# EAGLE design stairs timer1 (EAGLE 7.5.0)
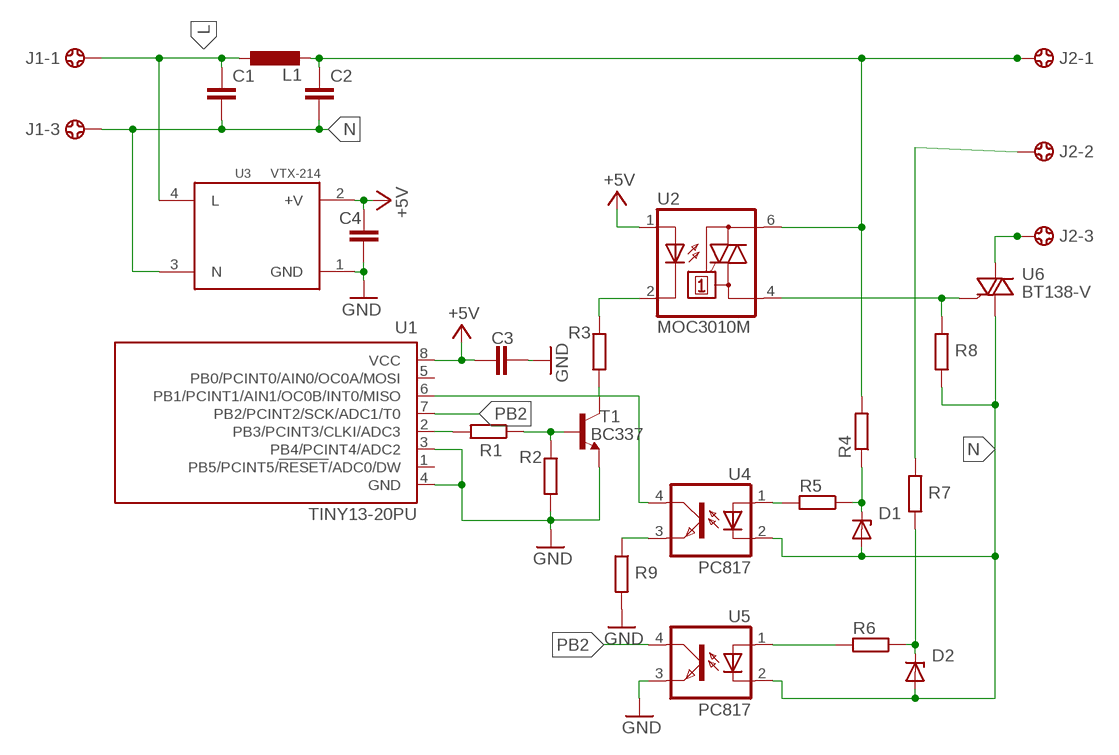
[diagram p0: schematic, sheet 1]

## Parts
C1  C-EU150-072X183  [C150-072X183]
C2  C-EU150-072X183  [C150-072X183]
C3  C-EUC1206  [C1206]
C4  C-EUC1206  [C1206]
D1  1N4728  [DO41Z10]
D2  1N4728  [DO41Z10]
J1  5202-03-N-02  [5202-03-N-02]
J2  5202-03-N-02  [5202-03-N-02]
L1  L-EUTJ8-U1  [TJ8-U1]
R1  R-EU_0204/7  [0204/7]
R2  R-EU_0204/7  [0204/7]
R3  R-EU_0204/7  [0204/7]
R4  R-EU_0617/22  [0617/22]
R5  R-EU_0204/7  [0204/7]
R6  R-EU_0204/7  [0204/7]
R7  R-EU_0617/22  [0617/22]
R8  R-EU_0204/7  [0204/7]
R9  R-EU_0204/7  [0204/7]
T1  BC337  [TO92]
U1  TINY13-20PU  [DIL08]
U2  MOC3010M  [DIL06]
U3  VTX-214  [VTX-214]
U4  PC817  [DIL04]
U5  PC817  [DIL04]
U6  BT138-V  [TO220BV]

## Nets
+5V: C3.1 C4.1 U1.8(VCC) U2.1(A) U3.2(+V)
GND: C3.2 C4.2 R2.2 R9.2 T1.1(E) U1.3(PB4/PCINT4/ADC2) U1.4(GND) U3.1(GND) U5.3(EMIT)
L: C1.1 J1.1 L1.1 U3.4(L)
N: C1.2 C2.2 D1.A D2.A J1.3 R8.2 U3.3(N) U4.2(C) U5.2(C) U6.T1(A1)
N$1: R1.2 U1.2(PB3/PCINT3/CLKI/ADC3)
N$2: R1.1 R2.1 T1.2(B)
N$3: C2.1 J2.1 L1.2 R4.2 U2.6(A2)
N$4: R5.2 U4.1(A)
N$5: R3.2 T1.3(C)
N$6: R3.1 U2.2(C)
N$7: D1.C R4.1 R5.1
N$8: R6.2 U5.1(A)
N$9: D2.C R6.1 R7.1
N$10: J2.2 R7.2
N$11: R8.1 U2.4(A1) U6.G
N$12: J2.3 U6.T2(A2)
N$13: R9.1 U4.3(EMIT)
PB1: U1.6(PB1/PCINT1/AIN1/OC0B/INT0/MISO) U4.4(COL)
PB2: U1.7(PB2/PCINT2/SCK/ADC1/T0) U5.4(COL)
Unconnected: J1.2 U1.1(PB5/PCINT5/!RESET!/ADC0/DW) U1.5(PB0/PCINT0/AIN0/OC0A/MOSI)

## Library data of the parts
C1-C4 = rcl:C-EU: CAPACITOR, European symbol
D1 D2 = diode:1N4728: Z DIODE
J1 J2 = con-ebyelectro:5202-03-N-02: Barrier Blocks Sreies 5202 Source: http://www.ebyelectro.com/PDF/5202-XX-N-02.pdf; OC_FARNELL: unknown; OC_NEWARK: unknown
L1 = rcl:L-EU: INDUCTOR, European symbol
R1-R9 = rcl:R-EU_: RESISTOR, European symbol
T1 = transistor:BC337: NPN TRANSISTOR
U1 = atmel:TINY13: 8-bit AVR Microcontroller with 1K Bytes In-System Programmable Flash Source: http://www.atmel.com/dyn/resources/prod_documents/2535S.pdf; MPN: ATTINY13-20PU; OC_FARNELL: 9171550; OC_NEWARK: 96K6521
U2 = optocoupler:MOC30*M: RANDOM-PHASE OPTOISOLATORS TRIAC DRIVER OUTPUT Source: http://www.fairchildsemi.com MOC3020-M.pdf; MF: FAIRCHILD SEMICONDUCTOR; MPN: MOC3010-M; OC_FARNELL: 1505423; OC_NEWARK: 72K8892
U3 = acdc:VTX-214: ACDC CONVERTER
U4 U5 = optocoupler:PC817: SHARP OPTO COUPLER; MPN: PC817X4J000F; OC_FARNELL: 9707727; OC_NEWARK: 97K7059
U6 = triac:BT138: TRIAC Source: http://www.semiconductors.philips.com BT138_SERIES_2.pdf

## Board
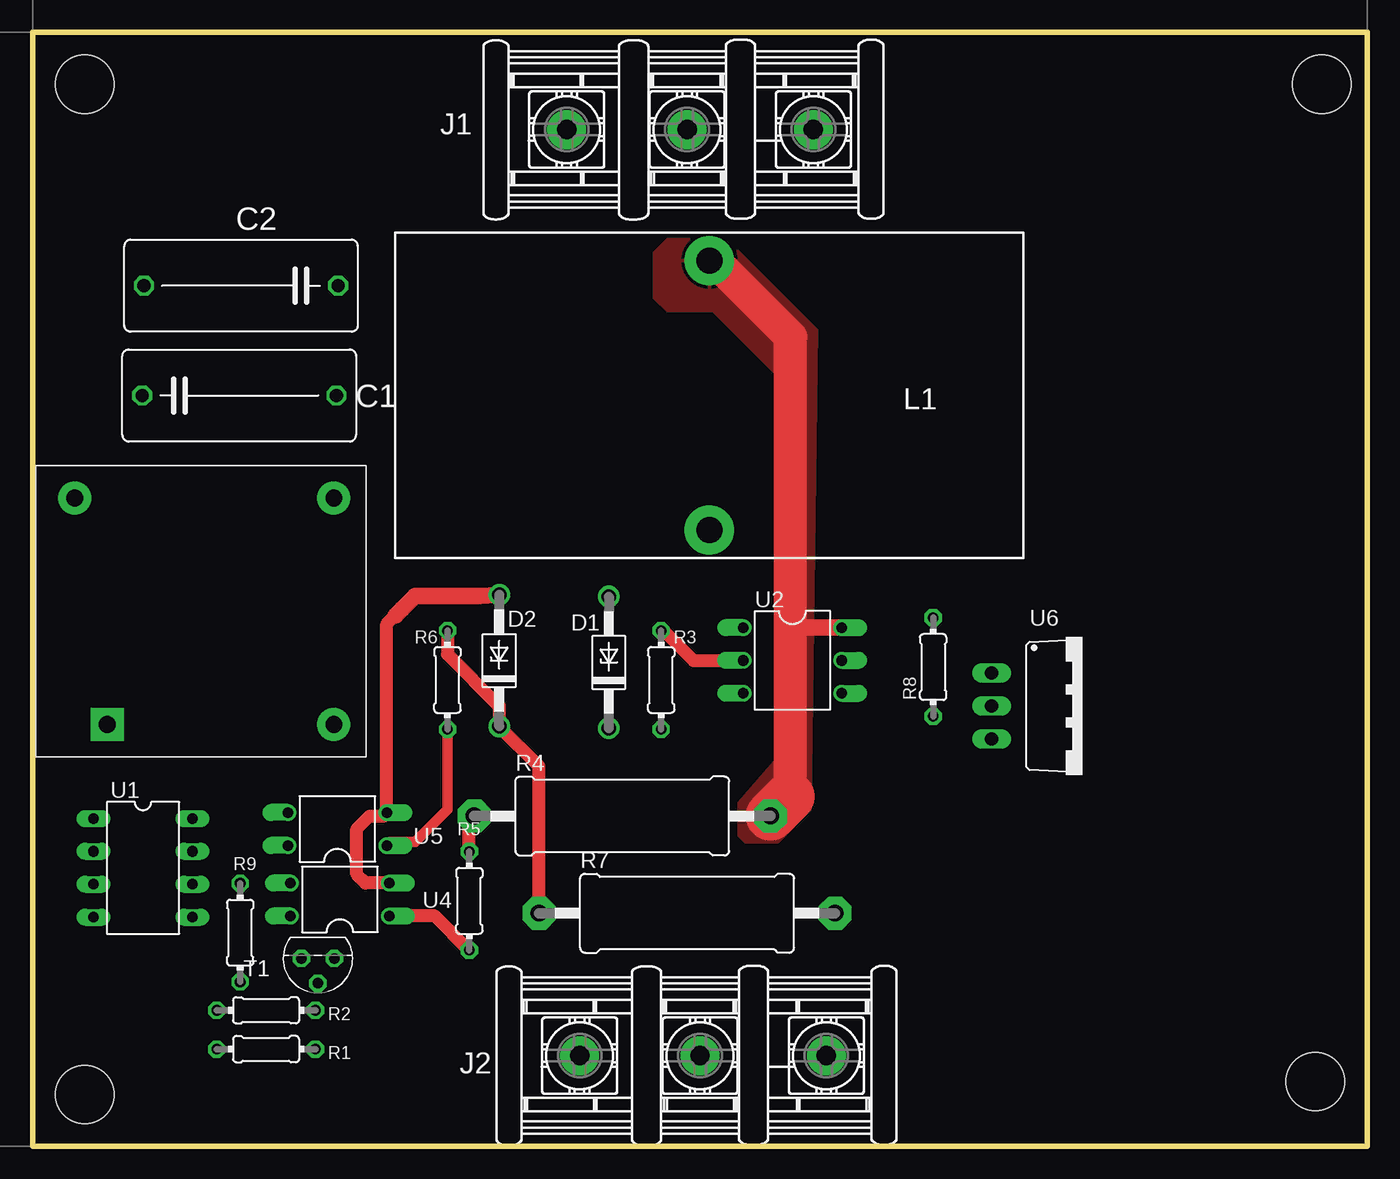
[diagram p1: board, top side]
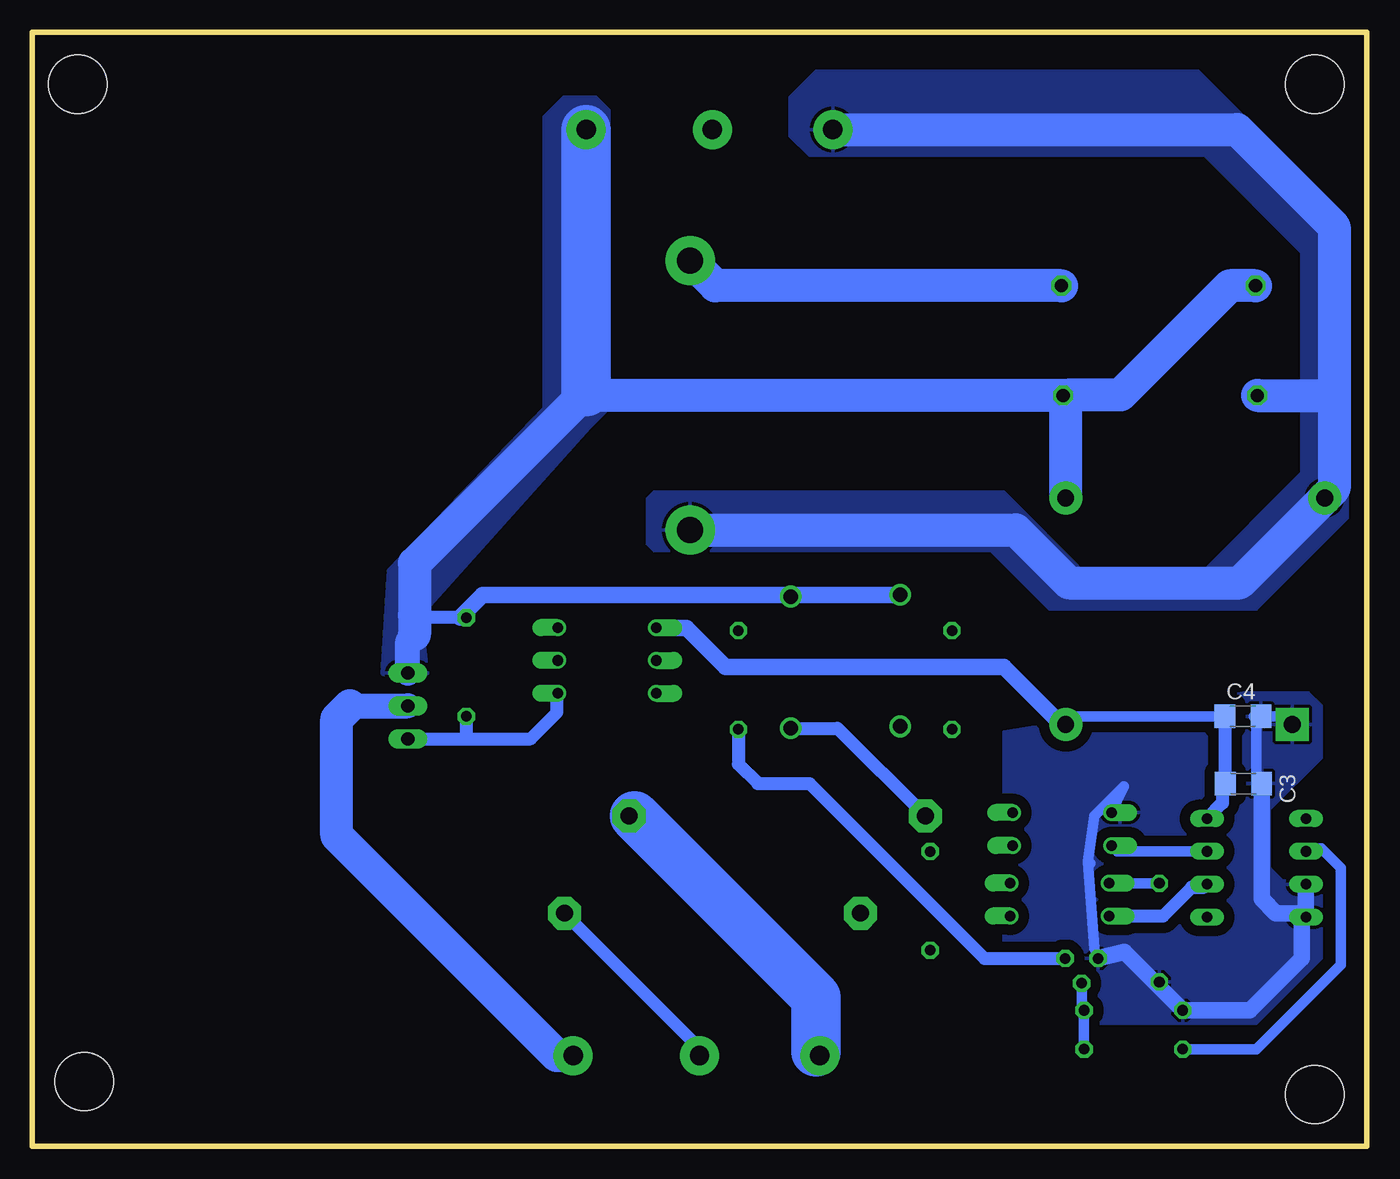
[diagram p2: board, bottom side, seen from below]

Size 103 x 86 mm. Coordinates in mm from the lower left corner, seen from the top.
Outline: 0,0 0,86 103,86 103,0 0,0
Copper layers (1*16): Top 0.035mm / dielectric 1.5mm / Bottom 0.035mm
Design rules "default": minimum track width 10mil, minimum drill 24mil, track to track 8mil, track to pad 8mil, pad to pad 8mil, via to via 8mil, smd to smd 8mil, copper to edge 40mil, drill to drill 8mil, minimum pad ring 10mil, minimum via ring 8mil, stop-mask expansion 4mil, vias tented up to drill 0mil, thermal gap 10mil
Holes 4.5 mm at 4,4 4,82 99.5,82 99,5

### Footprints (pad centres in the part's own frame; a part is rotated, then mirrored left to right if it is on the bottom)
C150-072X183 = drill 1.016 octagon: 1 -7.493,0; 2 7.493,0
C1206 = smd 1.6 x 1.8: 1 -1.4,0; 2 1.4,0
DO41Z10 = drill 1.118: A 5.08,0; C -5.08,0
5202-03-N-02 = drill 1.5 pad 3: 1 -9.29,0; 2 0,0; 3 9.75,0
TJ8-U1 = drill 2 pad 3.81: 1 -10.4,0; 2 10.4,0
0204/7 = drill 0.813 octagon: 1 -3.81,0; 2 3.81,0
0617/22 = drill 1.3 pad 2.54 octagon: 1 -11.43,0; 2 11.43,0
TO92 = drill 0.813 octagon: 1 1.27,0; 2 0,1.905; 3 -1.27,0
DIL08 = drill 0.813 long: 1 -3.81,-3.81; 2 -1.27,-3.81; 3 1.27,-3.81; 4 3.81,-3.81; 5 3.81,3.81; 6 1.27,3.81; 7 -1.27,3.81; 8 -3.81,3.81
DIL06 = drill 0.813 offset: 1 -2.54,-3.81; 2 0,-3.81; 3 2.54,-3.81; 4 2.54,3.81; 5 0,3.81; 6 -2.54,3.81
VTX-214 = drill 1.3 pad 2.54 square: 1 0,0 | drill 1.3 pad 2.54: 2 17.5,0; 3 17.5,17.5; 4 -2.5,17.5
DIL04 = drill 0.813 offset: 1 -1.27,-3.81; 2 1.27,-3.81; 3 1.27,3.81; 4 -1.27,3.81
TO220BV = drill 1.016 long: G 2.54,-6.985; T1 -2.54,-6.985; T2 0,-6.985

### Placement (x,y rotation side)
C1  15.93,57.97 0 top
C2  16.07,66.44 180 top
C3  9.5,28 0 bottom
C4  9.55,33.2 0 bottom
D1  44.46,37.36 90 top
D2  36,37.5 90 top
J1  50.5,78.5 0 top
J2  51.5,7 0 top
L1  52.22,57.98 90 top
R1  18,7.5 180 top
R2  18,10.5 180 top
R3  48.5,36 270 top
R4  45.5,25.5 0 top
R5  33.69,18.95 270 top
R6  32,36 270 top
R7  50.5,18 0 top
R8  69.5,37 90 top
R9  16,16.5 270 top
T1  22,14.5 180 top
U1  8.5,21.5 270 top
U2  58.63,37.51 270 top
U3  5.73,32.56 0 top
U4  23.7,19.06 90 top
U5  23.5,24.5 90 top
U6  81,34 270 top

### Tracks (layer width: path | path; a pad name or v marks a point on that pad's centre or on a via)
+5V
  Bottom 0.813: C4.1 22.59,33.2 U3.2 | C3.1 11.12,28
  Bottom 1.016: C3.1 10.9,33.15 C4.1 | 11.12,28 11.12,26.5 U1.8
  Bottom 1.27: U3.2 23.56,32.56 28,37 49.5,37 52.5,40 54.77,40 U2.1
GND
  Bottom 0.813: C4.2 6.37,33.2 U3.1 | U5.3 18.73,27.77 21,25.5 21.5,22 | 21.5,22 21,15.27 T1.1 | 21.33,21.83 21.5,22 | C4.2 6.2,33.2 6,33 | C4.2 8.7,33.2 8.5,33 8.5,28.4 C3.2
  Bottom 1.27: U1.4 5,17.38 5,14.5 9,10.5 R2.2 18.69,15 T1.1 | C3.2 8.1,19.1 7,18 5,18 U1.4 | U1.3 U1.4
  pour Bottom (isolate 0.813): 3.5,34 3.5,30 7.5,26 7.5,21.5 6.5,20.5 4,20.5 3.5,20 3.5,14.5 8.5,9.5 27,9.5 28,10.5 28,32 9.5,35 4.5,35
L
  Bottom 2.54: J1.1 10,78.5 2.5,71 2.5,58 | 2.5,58 2.5,50.79 U3.4 9.79,43.5 23,43.5 27.08,47.58 L1.1 | C1.1 2.53,57.97 2.5,58
  pour Bottom (isolate 1.016): 53,50.5 28,50.5 21.5,44 13,44 5,52 5,69 12.5,76.5 43,76.5 44.5,78 44.5,81 42.5,83 13,83 1.5,71.5 1.5,48.5 8.5,41.5 9,41.5 24.5,41.5 29,46 55,46 55.5,46.5 55.5,50 55,50.5
N
  Top 1.016: U4.2 25.67,20.33 25,21 25,24.5 26,25.5 27.04,25.5 U5.2 27.31,40.31 28.5,41.5
  Top 1.27: D2.A 35.92,42.58 34.5,42.5 29.5,42.5 28.5,41.5 28,41
  Bottom 1.016: D2.A 36.08,42.58 | R8.2 70,40.81 73.31,40.81 73.5,41
  Bottom 1.27: 44.32,42.58 D1.A | 44.32,42.58 68.23,42.58 70,40.81 | 36.08,42.58 44.32,42.58
  Bottom 1.93: U6.T1 74.02,38.98 73.5,39.5 | 60.25,57.75 60.5,58
  Bottom 2.54: C2.2 10.56,66.44 19,58 22.89,58 C1.2 | 60.25,58.25 60.5,58 73.5,45 73.5,41 73.5,39.5 | C1.2 60.03,57.97 60.25,57.75 | U3.3 23.23,57.78 C1.2
  Bottom 3.81: J1.3 60.25,58.25
  pour Bottom (isolate 1.27): 72.5,36.5 73,41 60,55.5 58.5,57 58.5,80 59.5,81 62,81 63.5,79.5 63.5,57 75.5,44.5 76,36.5 75,35.5 73.5,35.5
N$1
  Bottom 0.813: R1.2 8.5,7.5 2,14 2,21.5 3.5,23 4.46,23 U1.2
N$2
  Bottom 0.813: T1.2 22,10.69 R2.1 R1.1
N$3
  Top 1.27: U2.6 58.55,40.05 58.5,40
  Top 1.93: L1.2 52.62,68.38
  Top 2.54: 52.62,68.38 58.5,62.5 58.5,40 58.5,27 58.43,27
  Top 3.81: 58.43,27 R4.2
  Bottom 2.54: C2.1 50.28,66.44 L1.2 | R4.2 56.5,25.5 | 42.5,7.29 J2.1
  Bottom 3.81: 56.5,25.5 42.5,11.5 42.5,7.29
  pour Top (isolate 0.813): 49,70 53.5,70 60.5,63 60,26 57.5,23.5 55,23.5 54.5,24 54.5,26.5 57.5,30 57.5,59.5 52.5,64.5 49,64.5 48,65.5 48,69
N$4
  Top 1.016: R5.2 31.04,17.79 U4.1
N$5
  Bottom 1.016: R3.2 48.5,29.5 47,28 43,28 29.5,14.5 T1.3
N$6
  Top 1.016: R3.1 48.5,40 51,37.5 U2.2
N$7
  Top 1.016: R5.1 33.69,25.12 R4.1
  Bottom 1.016: D1.C 40.85,32.28 R4.1
N$8
  Top 0.813: R6.2 32,26 29.5,23.5 27.58,23.5 U5.1
N$9
  Top 1.016: R6.1 32,38 36,34 D2.C 39.07,29.35 R7.1
N$10
  Bottom 1.016: J2.2 51.5,7.57 R7.2
N$11
  Bottom 1.016: U6.G 69.5,31.46 | 69.5,31.46 64.54,31.46 62.5,33.5 62.5,34.91 U2.4 | R8.1 69.5,31.46
N$12
  Bottom 1.93: 78.5,34 U6.T2
  Bottom 2.54: J2.3 62.5,7 79.5,24 79.5,33 78.5,34
N$13
  Bottom 0.813: R9.1 19.87,20.31 U4.3
PB1
  Bottom 1.016: U4.4 15.71,17.79 13.5,20 12.54,20 U1.6
PB2
  Bottom 0.813: U1.7 19.23,22.77 U5.4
